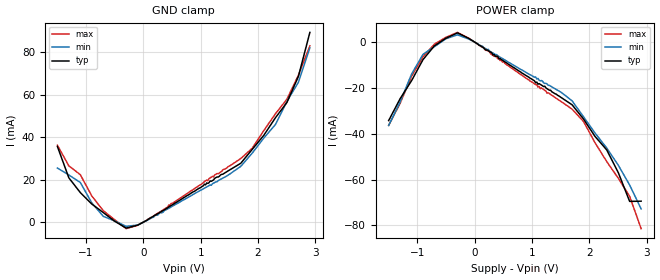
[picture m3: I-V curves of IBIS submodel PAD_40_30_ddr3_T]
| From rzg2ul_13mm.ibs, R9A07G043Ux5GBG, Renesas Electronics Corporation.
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[Submodel]  PAD_40_30_ddr3_T
Submodel_type Dynamic_clamp
[GND Clamp]
| Voltage   I(typ)   I(min)   I(max)
-1.5V     35.59mA    25.45mA    36.2mA
-1.3V     20.84mA    22.19mA    26.46mA
-1.1V     13.91mA    18.66mA    22.34mA
-900mV    8.532mA    9.057mA    12.33mA
-700mV    4.527mA    2.751mA    5.404mA
-300mV    -2.766mA   -1.958mA   -3.046mA
-100mV    -1.393mA   -1.347mA   -1.479mA
1.7V      27.71mA    26.26mA    29.94mA
2.305V    49.13mA    45.94mA    51mA
2.505V    56.31mA    56.83mA    57.86mA
2.705V    68.56mA    65.81mA    69.11mA
2.905V    89.24mA    82.01mA    82.93mA
[POWER Clamp]
| Voltage   I(typ)   I(min)   I(max)
-1.5V     -34.26mA   -36.37mA   -36.38mA
-1.1V     -16.84mA   -13.96mA   -14.93mA
-900mV    -7.638mA   -5.331mA   -6.411mA
-700mV    -1.605mA   -1.975mA   -857.8uA
-300mV    4.018mA    3.166mA    4.225mA
240mV     -3.781mA   -3.2mA     -3.965mA
1.7V      -27.36mA   -25.63mA   -29.26mA
1.9V      -33.59mA   -32.6mA    -34.65mA
2.305V    -47.07mA   -46.25mA   -52.16mA
2.505V    -56.88mA   -53.67mA   -59.36mA
2.705V    -69.54mA   -62.4mA    -67.34mA
2.905V    -69.43mA   -72.8mA    -81.43mA
